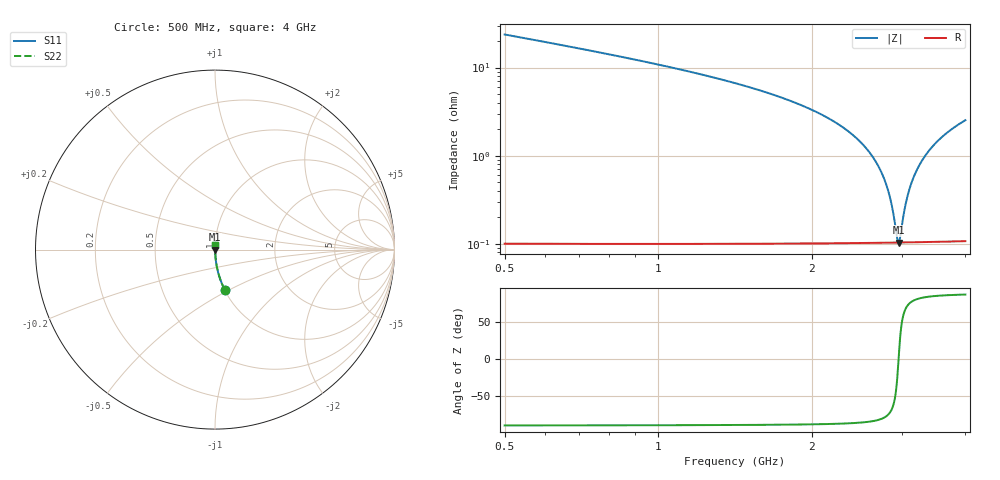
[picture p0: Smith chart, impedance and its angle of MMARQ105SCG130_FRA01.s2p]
! MMARQ105SCG130_FRA01  S-PARAMETER MODEL  ( General Type )
! Model Generated by TAIYO YUDEN Corporation (http://www.ty-top.com)
! Version 1.0
! TAIYO YUDEN Control No. 200326
! Copyright(c) 2020 TAIYO YUDEN CO.,LTD. All Rights Reserved.
! Product Description (link to TY-COMPAS)
! https://ds.yuden.co.jp/TYCOMPAS/or/detail?pn=MMARQ105SCG130JFRA01&u=M
! Products Name : Multilayer Ceramic Capacitors
! Characteristics :
!  Capacitance : 13 pF , Rated Voltage : 250V , TCC : CG / C0G
!  Case Size : 1.0 x 0.5 / 0.039 x 0.02 [mm/inch] , Thickness : 0.5 / 0.02 [mm/inch]
!  (Conditions: Temperature = 25 degC , DC Bias Current/Voltage = 0A / 0V)
! External Node Assignments :
!  1  o---| |---o  2
! GND o---------o GND
! Frequency Range : 500MHz  -  4GHz  [ 401 STEP ]
# MHz S RI R 50
! Freq[MHz].  S11 Real  S11 Imag  S21 Real  S21 Imag  S12 Real  S12 Imag  S22 Real  S22 Imag
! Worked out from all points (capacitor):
!   401 points, 500 MHz to 4 GHz, reference 50 ohm
!   read as one part in series: C = 13 pF near 517.5 MHz
!   lowest |Z| = 104 mohm at 2.959 GHz (marker M1)
!   series resonance near 2.959 GHz, so ESL is about 220 pH
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500  0.0542 -0.2243  0.9458 0.2243  0.9458 0.2243  0.0542 -0.2243
762.5  0.0228 -0.1461  0.9772 0.1461  0.9772 0.1461  0.0228 -0.1461
1086.25  0.0104 -0.0962  0.9896 0.0962  0.9896 0.0962  0.0104 -0.0962
1672.5  0.00346 -0.0495  0.9965 0.0495  0.9965 0.0495  0.00346 -0.0495
1996.25  0.00212 -0.0332  0.9979 0.0332  0.9979 0.0332  0.00212 -0.0332
2250  0.00154 -0.0228  0.9985 0.0228  0.9985 0.0228  0.00154 -0.0228
2460  0.00126 -0.0153  0.9987 0.0153  0.9987 0.0153  0.00126 -0.0153
2626.25  0.00112 -0.00985  0.9989 0.00985  0.9989 0.00985  0.00112 -0.00985
2748.75  0.00107 -0.00607  0.9989 0.00607  0.9989 0.00607  0.00107 -0.00607
2836.25  0.00104 -0.00349  0.999 0.00349  0.999 0.00349  0.00104 -0.00349
2880  0.00104 -0.00222  0.999 0.00222  0.999 0.00222  0.00104 -0.00222
2941.25  0.00104 -0.000489  0.999 0.000489  0.999 0.000489  0.00104 -0.000489
2958.75  0.00104 1.82e-07  0.999 -1.82e-07  0.999 -1.82e-07  0.00104 1.82e-07
2976.25  0.00104 0.000486  0.999 -0.000486  0.999 -0.000486  0.00104 0.000486
3028.75  0.00104 0.00193  0.999 -0.00193  0.999 -0.00193  0.00104 0.00193
3063.75  0.00105 0.00288  0.999 -0.00288  0.999 -0.00288  0.00105 0.00288
3098.75  0.00105 0.00381  0.9989 -0.00381  0.9989 -0.00381  0.00105 0.00381
3142.5  0.00107 0.00497  0.9989 -0.00497  0.9989 -0.00497  0.00107 0.00497
3265  0.00111 0.00813  0.9989 -0.00813  0.9989 -0.00813  0.00111 0.00813
3422.5  0.0012 0.012  0.9988 -0.012  0.9988 -0.012  0.0012 0.012
3676.25  0.00139 0.018  0.9986 -0.018  0.9986 -0.018  0.00139 0.018
4000  0.00171 0.0252  0.9983 -0.0252  0.9983 -0.0252  0.00171 0.0252
